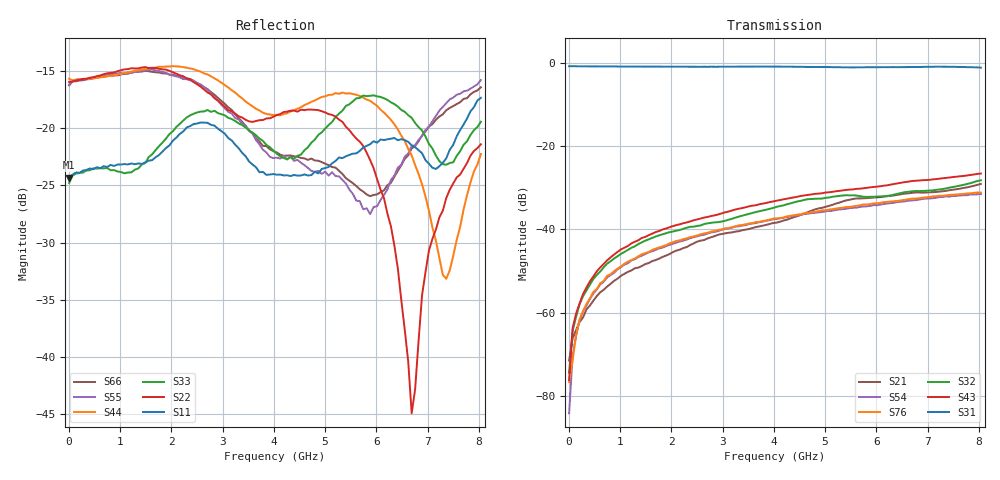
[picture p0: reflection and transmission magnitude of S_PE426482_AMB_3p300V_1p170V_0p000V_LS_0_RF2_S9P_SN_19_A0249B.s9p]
! Device ID: PE426482
! File Path: z:\PE426482\Final Char Data\room\AMB\3p300\LS_0_RF2\PE426482_AMB_3p300V_1p170V_0p000V_LS_0_RF2_S9P_SN_19_A0249B.s9p
! Serial: 19
! Lot: A0249B
! Temp: AMB
! VDD: 3.300
! VSS: 0.000
! Control_Hi: 1.170
! Control_Lo: 0.000
! Logic State: LS_0_RF2
! Port 1:
! Port 2:
! Port 3:
! Port 4:
! Port 5:
! Port 6:
! Port 7:
! Port 8:
! Port 9:
! ThroughPath:1-3
! IDD: 0.000107603
! ISS/IDD2: -3.33e-008
! IDMM3/IDD3: -2.154e-007
! Comment:
#  Hz  S  RI  R  50
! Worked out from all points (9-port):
!   120 points, 10 MHz to 8.037 GHz, reference 50 ohm
!   strongest paths, dB at 10 MHz, 2.034 GHz, 4.057 GHz, 6.08 GHz, 8.037 GHz:
!     S31: -0.8, -0.9, -0.9, -1.0, -1.1
!     S43: -76.2, -39.2, -33.1, -29.6, -26.6
!     S32: -74.5, -40.5, -34.6, -32.1, -28.2
!     S76: -76.7, -43.1, -37.4, -33.6, -31.2
!     S54: -84.2, -43.5, -37.5, -34.0, -31.5
!     S21: -71.6, -45.5, -38.4, -32.2, -29.1
!   lowest |S11| = -24.3 dB at 10 MHz (marker M1), VSWR 1.13, Z = 56.5 + j0.0823 ohm
!   |S11| at or under -10 dB: start of sweep to end of sweep
